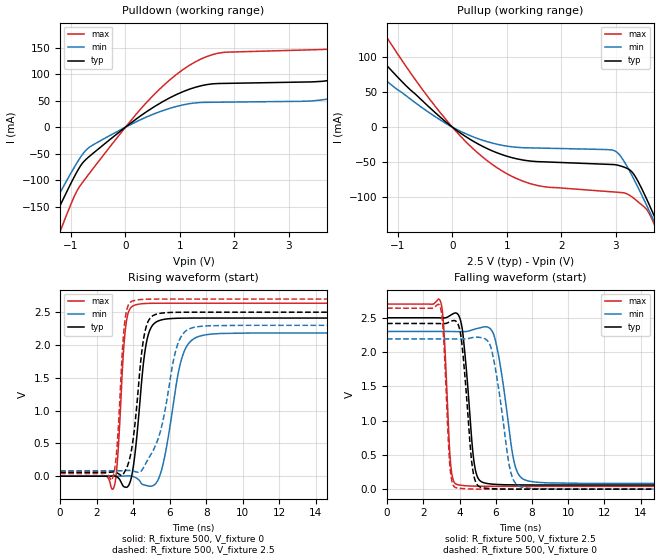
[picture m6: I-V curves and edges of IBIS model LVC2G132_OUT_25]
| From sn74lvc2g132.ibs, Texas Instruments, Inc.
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[Model]   LVC2G132_OUT_25
Model_type  Output
Vref =   0
Rref =   500
Cref =   30p
Vmeas =   1.25
| variable   typ   min   max
C_comp   9.81pF   6.17pF   14.72pF
| C_pullup   9.66pF   6.17pF   11.33pF
| C_pulldown   9.96pF   6.66pF   14.72pF
[Temperature Range]   40   100   -40
| Ambient temperature   25   85   -40
[Voltage range]   2.5   2.3   2.7
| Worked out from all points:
|   slope of the pulldown table from 0 to 0.375 V, typ, clamps not added: 13.3 ohm
|   slope of the pullup table from 0 to 0.375 V, typ, clamps not added: 19 ohm
|   rising waveform, R_fixture 500, V_fixture 0: 20-80 % time 505ps typ, 791ps min, 320ps max; typ from 0 V to 2.41 V
|   falling waveform, R_fixture 500, V_fixture 2.5: 20-80 % time 449ps typ, 702ps min, 280ps max; typ from 2.5 V to 0.061 V
|   rising waveform, R_fixture 500, V_fixture 2.5: 20-80 % time 535ps typ, 973ps min, 327ps max; typ from 0.061 V to 2.5 V
|   falling waveform, R_fixture 500, V_fixture 0: 20-80 % time 436ps typ, 704ps min, 278ps max; typ from 2.42 V to 0 V
[Pulldown]
| LVC2G132_OUT_25
|   Voltage   I(typ)   I(min)   I(max)
-5.5V     -1.06A     -941.4mA   -1.275A
-1.52V    -217.1mA   -184.1mA   -281.2mA
-1.26V    -160.6mA   -134.6mA   -212.3mA
-665mV    -55.38mA   -37.96mA   -87.52mA
385mV     28.96mA    19.04mA    46.35mA
1.275V    74.94mA    45.66mA    122.7mA
3.82V     89.63mA    55.12mA    148.2mA
5.34V     157.4mA    105.8mA    232mA
5.91V     188.7mA    52.55mA    283.4mA
6.525V    93.54mA    53.06mA    299.5mA
7.555V    94.08mA    54.03mA    161.4mA
11V       99.63mA    57.49mA    169.6mA
[Pullup]
| LVC2G132_OUT_25
|   Voltage   I(typ)   I(min)   I(max)
-5.5V     533.4mA    418.6mA    746.4mA
-2.335V   192.2mA    147mA      274.9mA
-1.875V   147.9mA    112.2mA    212.9mA
-1.315V   97.38mA    72.9mA     141.5mA
-225mV    14.47mA    10.42mA    20.98mA
735mV     -33.88mA   -22.76mA   -53.28mA
1.56V     -49.18mA   -29.79mA   -83.17mA
2.98V     -53.48mA   -33.7mA    -92.52mA
3.325V    -66.27mA   -72.72mA   -100.9mA
3.755V    -135mA     -142.5mA   -147.1mA
3.835V    -149.5mA   -156.2mA   -162.8mA
11V       -1.609A    -1.492A    -1.841A
[Ramp]
| LVC2G132_OUT_25
| variable   typ   min   max
dV/dt_r   1.55/5.43E-10   1.40/8.49E-10   1.70/3.51E-10
dV/dt_f   1.51/4.67E-10   1.37/7.34E-10   1.64/2.97E-10
R_load = 500
[Rising Waveform]
| LVC2G132_OUT_25
R_fixture =   500
C_fixture =   0
L_fixture =   0
V_fixture =   0
V_fixture_min = 0
V_fixture_max = 0
|   Time   V(typ)   V(min)   V(max)
0s        125.3pV    6.247nV    2.314nV
2.93ns    4.698mV    -102.5uV   -179.5mV
3.605ns   -169mV     3.881mV    2.312V
4.24ns    723.7mV    -38.64mV   2.619V
4.62ns    1.853V     -135.5mV   2.632V
5ns       2.276V     -152.8mV   2.635V
5.625ns   2.387V     170.6mV    2.637V
6.725ns   2.409V     1.852V     2.637V
7.875ns   2.411V     2.151V     2.637V
45ns      2.411V     2.183V     2.637V
[Falling Waveform]
| LVC2G132_OUT_25
R_fixture =   500
C_fixture =   0
L_fixture =   0
V_fixture =   2.5
V_fixture_min = 2.3
V_fixture_max = 2.7
|   Time   V(typ)   V(min)   V(max)
0s        2.5V       2.3V       2.7V
2.935ns   2.498V     2.3V       2.751V
3.51ns    2.537V     2.3V       372.7mV
3.9ns     2.554V     2.298V     64.78mV
4.825ns   354.6mV    2.333V     43.99mV
5.41ns    88.97mV    2.369V     42.17mV
6.005ns   69.6mV     2.142V     41.7mV
7.075ns   62.37mV    334.2mV    41.54mV
7.82ns    61.42mV    117.5mV    41.53mV
45ns      60.93mV    83.64mV    41.46mV
[Rising Waveform]
| LVC2G132_OUT_25
R_fixture =   500
C_fixture =   0
L_fixture =   0
V_fixture =   2.5
V_fixture_min = 2.3
V_fixture_max = 2.7
|   Time   V(typ)   V(min)   V(max)
0s        60.91mV    83.6mV     41.45mV
2.87ns    64.2mV     83.55mV    -28.78mV
3.11ns    52.33mV    83.29mV    428mV
3.55ns    76.92mV    86.65mV    2.374V
4.12ns    854.9mV    69.6mV     2.682V
4.505ns   1.971V     103.1mV    2.695V
4.86ns    2.381V     280.7mV    2.698V
6.44ns    2.498V     2.012V     2.7V
7.39ns    2.5V       2.273V     2.7V
45ns      2.5V       2.3V       2.7V
[Falling Waveform]
| LVC2G132_OUT_25
R_fixture =   500
C_fixture =   0
L_fixture =   0
V_fixture =   0
V_fixture_min = 0
V_fixture_max = 0
|   Time   V(typ)   V(min)   V(max)
0s        2.416V     2.191V     2.64V
2.935ns   2.415V     2.192V     2.661V
3.475ns   2.443V     2.191V     319.2mV
3.81ns    2.448V     2.19V      19.38mV
4.125ns   2.135V     2.189V     9.725mV
4.73ns    284.9mV    2.212V     2.137mV
5.225ns   23.94mV    2.209V     723uV
6.85ns    1.01mV     227.1mV    92.73uV
7.505ns   387.1uV    24.86mV    76.33uV
45ns      25.46uV    41.25uV    14.13uV
